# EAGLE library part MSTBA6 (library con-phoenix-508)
PHOENIX
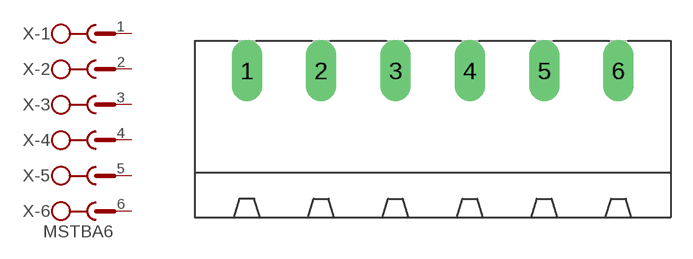
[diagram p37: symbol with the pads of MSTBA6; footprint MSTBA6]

Designator prefix X; gates -1=SK -2=SK -3=SK -4=SK -5=SK -6=SKV

## MSTBA6 (MF: FARNELL; MPN: 1757284; OC_FARNELL: 3705213; OC_NEWARK: 71C4165)  [MSTBA6]
1  -1:1  pas
2  -2:1  pas
3  -3:1  pas
4  -4:1  pas
5  -5:1  pas
6  -6:1  pas

## Footprint MSTBA6 (pad centres in mm)
PHOENIX
drill 1.397 long: 1 -12.7,5.08; 2 -7.62,5.08; 3 -2.54,5.08; 4 2.54,5.08; 5 7.62,5.08; 6 12.7,5.08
